FUNCTION "FC_GRP_43" : VOID
TITLE =GROUP =43
{ S7_language := '9(1) Angielski (Stany Zjednoczone)  11.01.2022  09:45:15' }
VERSION : 0.1


VAR_TEMP
  CL : "UDT_CABINET";	//CABINET LOCAL
  CR : "UDT_CABINET";	//CABINET REMOTE
  RelError : BOOL ;	//ERROR RELEASE
  RelErrorCL : BOOL ;	//ERROR RELEASE FROM CABINET LOCAL
  RelErrorCR : BOOL ;	//ERROR RELEASE FROM CABINET REMOTE
  RelControl : BOOL ;	//CONTROL RELEASE
  RelControlCL : BOOL ;	//CONTROL RELEASE FROM CABINET LOCAL
  RelControlCR : BOOL ;	//CONTROL RELEASE FROM CABINET REMOTE
  ErrorConfirm : BOOL ;	//ERROR CONFIRM
  AutoOn : BOOL ;	//AUTOMATIC ON
  AutoOff : BOOL ;	//AUTOMATIC OFF
  RelAuto : BOOL ;	//AUTOMATIC RELEASE
  LAMP_ON : BOOL ;
  TempSetpoint : REAL ;
END_VAR
BEGIN
NETWORK
TITLE =GLOBAL SIGNALS
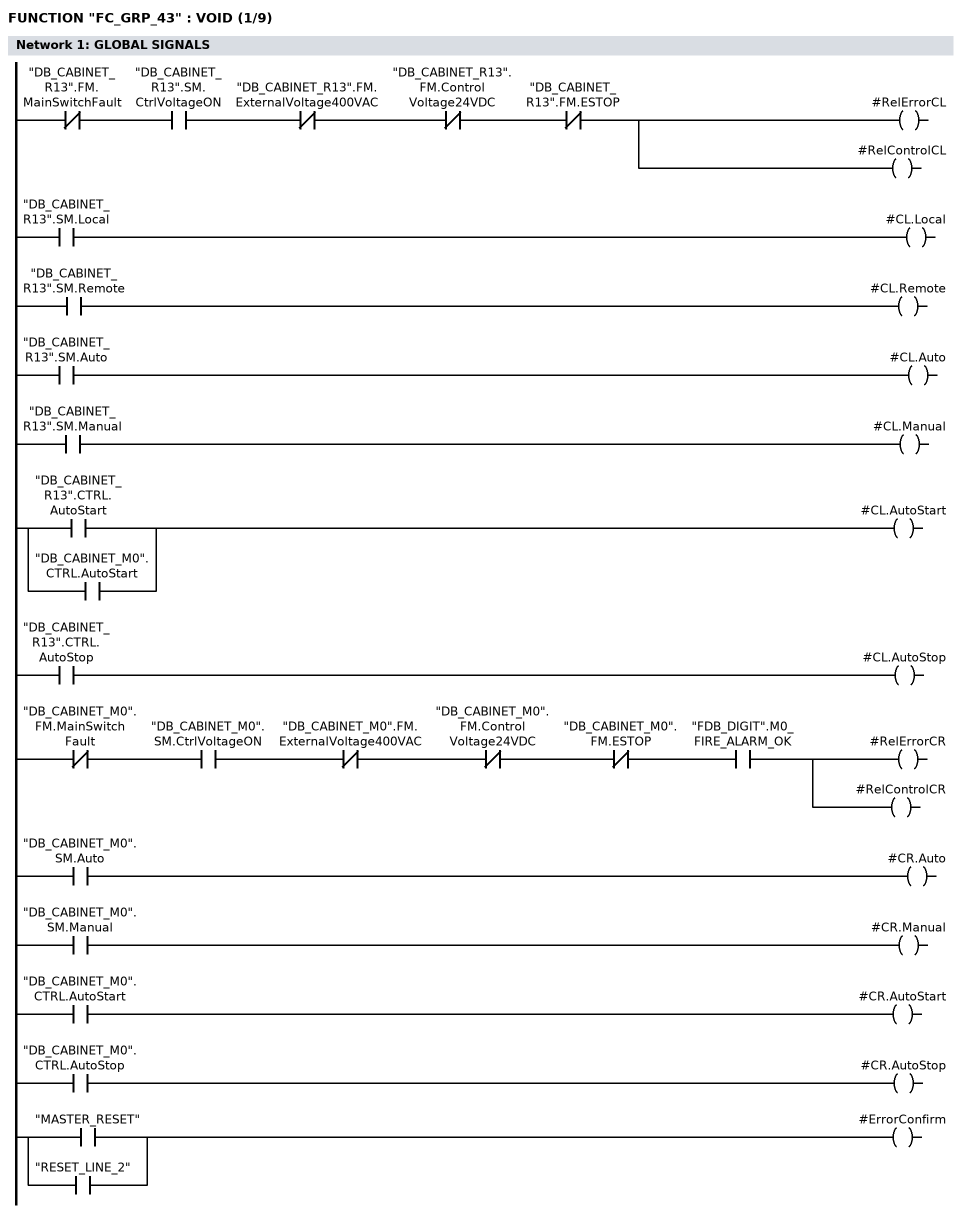
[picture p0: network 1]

//LOCAL
      UN    "DB_CABINET_R13".FM.MainSwitchFault;
      U     "DB_CABINET_R13".SM.CtrlVoltageON;
      UN    "DB_CABINET_R13".FM.ExternalVoltage400VAC;
      UN    "DB_CABINET_R13".FM.ControlVoltage24VDC;
      UN    "DB_CABINET_R13".FM.ESTOP;
      =     #RelErrorCL;
      =     #RelControlCL;

      U     "DB_CABINET_R13".SM.Local;
      =     #CL.Local;
      U     "DB_CABINET_R13".SM.Remote;
      =     #CL.Remote;
      U     "DB_CABINET_R13".SM.Auto;
      =     #CL.Auto;
      U     "DB_CABINET_R13".SM.Manual;
      =     #CL.Manual;
      U     "DB_CABINET_R13".CTRL.AutoStart;
      O     "DB_CABINET_M0".CTRL.AutoStart;
      =     #CL.AutoStart;
      U     "DB_CABINET_R13".CTRL.AutoStop;
      =     #CL.AutoStop;


//REMOTE
      UN    "DB_CABINET_M0".FM.MainSwitchFault;
      U     "DB_CABINET_M0".SM.CtrlVoltageON;
      UN    "DB_CABINET_M0".FM.ExternalVoltage400VAC;
      UN    "DB_CABINET_M0".FM.ControlVoltage24VDC;
//      UN    "DB_CABINET_M0".FM.ControlVoltage230VAC_MS
      UN    "DB_CABINET_M0".FM.ESTOP;
      U     "FDB_DIGIT".M0_FIRE_ALARM_OK;
      =     #RelErrorCR;
      =     #RelControlCR;

      U     "DB_CABINET_M0".SM.Auto;
      =     #CR.Auto;
      U     "DB_CABINET_M0".SM.Manual;
      =     #CR.Manual;
      U     "DB_CABINET_M0".CTRL.AutoStart;
      =     #CR.AutoStart;
      U     "DB_CABINET_M0".CTRL.AutoStop;
      =     #CR.AutoStop;


      U     "MASTER_RESET";
      O     "RESET_LINE_2";
      =     #ErrorConfirm;

NETWORK
TITLE =GLOBAL SIGNALS - GROUP GENERAL ERROR AND WARNING
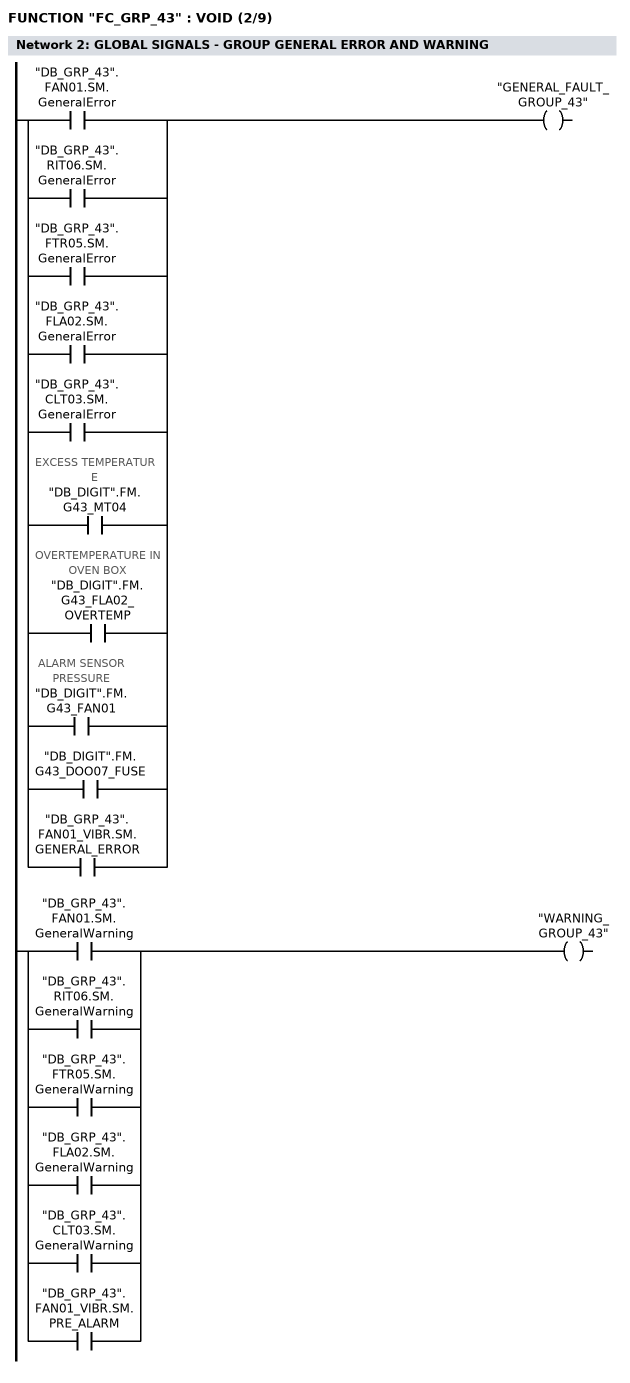
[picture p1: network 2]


      U     "DB_GRP_43".FAN01.SM.GeneralError;
      O     "DB_GRP_43".RIT06.SM.GeneralError;
      O     "DB_GRP_43".FTR05.SM.GeneralError;
      O     "DB_GRP_43".FLA02.SM.GeneralError;
      O     "DB_GRP_43".CLT03.SM.GeneralError;
      O     "DB_DIGIT".FM.G43_MT04; //EXCESS TEMPERATURE
      O     "DB_DIGIT".FM.G43_FLA02_OVERTEMP; //OVERTEMPERATURE IN OVEN BOX
      O     "DB_DIGIT".FM.G43_FAN01; //ALARM SENSOR PRESSURE
      O     "DB_DIGIT".FM.G43_DOO07_FUSE;
      O     "DB_GRP_43".FAN01_VIBR.SM.GENERAL_ERROR;
      =     "GENERAL_FAULT_GROUP_43";

      U     "DB_GRP_43".FAN01.SM.GeneralWarning;
      O     "DB_GRP_43".RIT06.SM.GeneralWarning;
      O     "DB_GRP_43".FTR05.SM.GeneralWarning;
      O     "DB_GRP_43".FLA02.SM.GeneralWarning;
      O     "DB_GRP_43".CLT03.SM.GeneralWarning;
      O     "DB_GRP_43".FAN01_VIBR.SM.PRE_ALARM;
      =     "WARNING_GROUP_43";


NETWORK
TITLE =RELEASE CONTROL
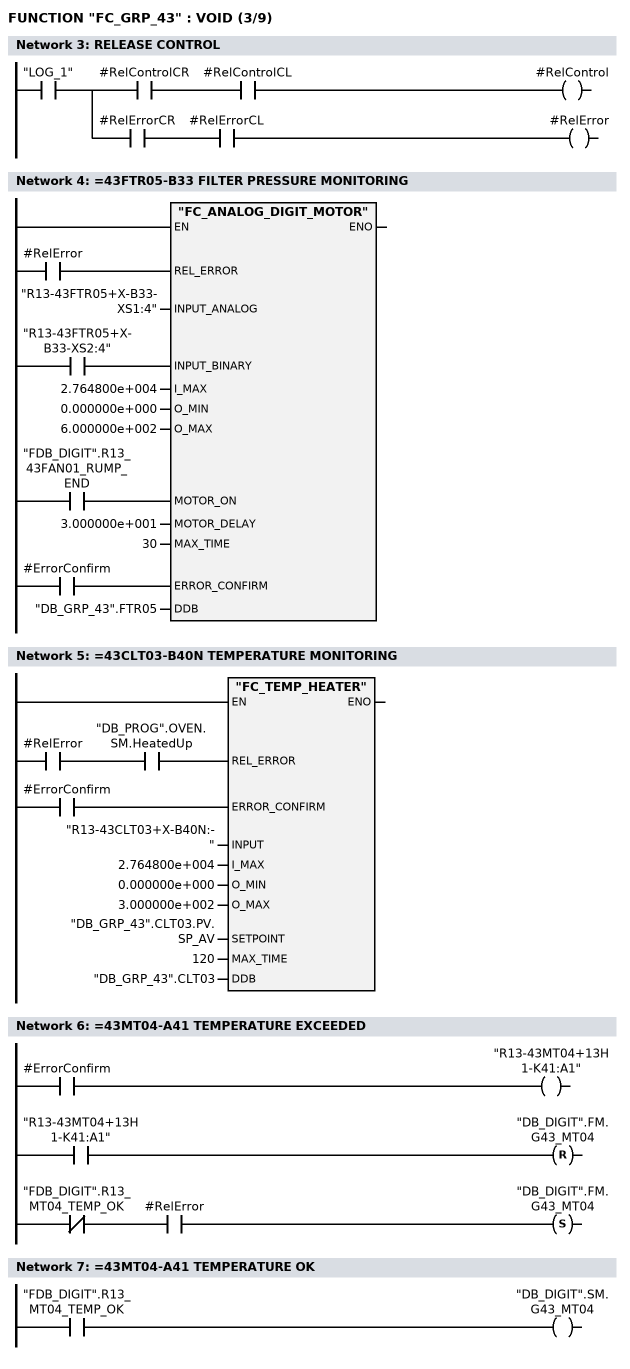
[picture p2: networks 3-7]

      U     "LOG_1";
      =     L     10.0;
      U     L     10.0;
      U     #RelControlCR;
      U     #RelControlCL;
      =     #RelControl;
      U     L     10.0;
      U     #RelErrorCR;
      U     #RelErrorCL;
      =     #RelError;
NETWORK
TITLE ==43FTR05-B33 FILTER PRESSURE MONITORING

      U     #RelError;
      =     L     10.0;
      BLD   103;
      U     "R13-43FTR05+X-B33-XS2:4";
      =     L     10.1;
      BLD   103;
      U     "FDB_DIGIT".R13_43FAN01_RUMP_END;
      =     L     10.2;
      BLD   103;
      U     #ErrorConfirm;
      =     L     10.3;
      BLD   103;
      CALL "FC_ANALOG_DIGIT_MOTOR" (
           REL_ERROR                := L     10.0,
           INPUT_ANALOG             := "R13-43FTR05+X-B33-XS1:4",
           INPUT_BINARY             := L     10.1,
           I_MAX                    := 2.764800e+004,
           O_MIN                    := 0.000000e+000,
           O_MAX                    := 6.000000e+002,
           MOTOR_ON                 := L     10.2,
           MOTOR_DELAY              := 3.000000e+001,
           MAX_TIME                 := 30,
           ERROR_CONFIRM            := L     10.3,
           DDB                      := "DB_GRP_43".FTR05);
      NOP   0;
NETWORK
TITLE ==43CLT03-B40N TEMPERATURE MONITORING

      U     #RelError;
      U     "DB_PROG".OVEN.SM.HeatedUp;
      =     L     10.0;
      BLD   103;
      U     #ErrorConfirm;
      =     L     10.1;
      BLD   103;
      CALL "FC_TEMP_HEATER" (
           REL_ERROR                := L     10.0,
           ERROR_CONFIRM            := L     10.1,
           INPUT                    := "R13-43CLT03+X-B40N:-",
           I_MAX                    := 2.764800e+004,
           O_MIN                    := 0.000000e+000,
           O_MAX                    := 3.000000e+002,
           SETPOINT                 := "DB_GRP_43".CLT03.PV.SP_AV,
           MAX_TIME                 := 120,
           DDB                      := "DB_GRP_43".CLT03);
      NOP   0;
NETWORK
TITLE ==43MT04-A41 TEMPERATURE EXCEEDED

      U     #ErrorConfirm;
      =     "R13-43MT04+13H1-K41:A1";
      U     "R13-43MT04+13H1-K41:A1";
      R     "DB_DIGIT".FM.G43_MT04;
      UN    "FDB_DIGIT".R13_MT04_TEMP_OK;
      U     #RelError;
      S     "DB_DIGIT".FM.G43_MT04;
      NOP   0;
NETWORK
TITLE ==43MT04-A41 TEMPERATURE OK

      U     "FDB_DIGIT".R13_MT04_TEMP_OK;
      =     "DB_DIGIT".SM.G43_MT04;
NETWORK
TITLE ==43DOO07-F1.1 ACCESS DOOR ERROR
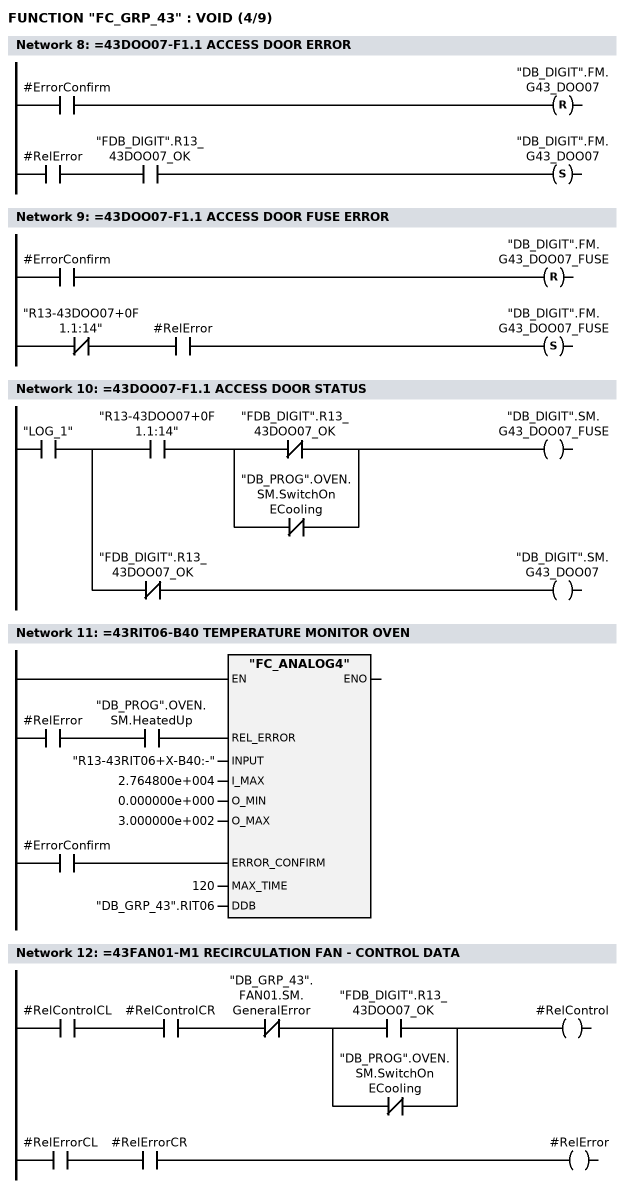
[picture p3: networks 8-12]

      U     #ErrorConfirm;
      R     "DB_DIGIT".FM.G43_DOO07;
      U     #RelError;
      U     "FDB_DIGIT".R13_43DOO07_OK;
      S     "DB_DIGIT".FM.G43_DOO07;
      NOP   0;
NETWORK
TITLE ==43DOO07-F1.1 ACCESS DOOR FUSE ERROR

      U     #ErrorConfirm;
      R     "DB_DIGIT".FM.G43_DOO07_FUSE;
      UN    "R13-43DOO07+0F1.1:14";
      U     #RelError;
      S     "DB_DIGIT".FM.G43_DOO07_FUSE;
      NOP   0;
NETWORK
TITLE ==43DOO07-F1.1 ACCESS DOOR STATUS

      U     "LOG_1";
      =     L     10.0;
      U     L     10.0;
      U     "R13-43DOO07+0F1.1:14";
      U(    ;
      ON    "FDB_DIGIT".R13_43DOO07_OK;
      ON    "DB_PROG".OVEN.SM.SwitchOnECooling;
      )     ;
      =     "DB_DIGIT".SM.G43_DOO07_FUSE;
      U     L     10.0;
      UN    "FDB_DIGIT".R13_43DOO07_OK;
      =     "DB_DIGIT".SM.G43_DOO07;
NETWORK
TITLE ==43RIT06-B40 TEMPERATURE MONITOR OVEN

      U     #RelError;
      U     "DB_PROG".OVEN.SM.HeatedUp;
      =     L     10.0;
      BLD   103;
      U     #ErrorConfirm;
      =     L     10.1;
      BLD   103;
      CALL "FC_ANALOG4" (
           REL_ERROR                := L     10.0,
           INPUT                    := "R13-43RIT06+X-B40:-",
           I_MAX                    := 2.764800e+004,
           O_MIN                    := 0.000000e+000,
           O_MAX                    := 3.000000e+002,
           ERROR_CONFIRM            := L     10.1,
           MAX_TIME                 := 120,
           DDB                      := "DB_GRP_43".RIT06);
      NOP   0;
NETWORK
TITLE ==43FAN01-M1 RECIRCULATION FAN - CONTROL DATA

      U     #RelControlCL;
      U     #RelControlCR;
      UN    "DB_GRP_43".FAN01.SM.GeneralError;
      U(    ;
      O     "FDB_DIGIT".R13_43DOO07_OK;
      ON    "DB_PROG".OVEN.SM.SwitchOnECooling;
      )     ;
      =     #RelControl;


      U     #RelErrorCL;
      U     #RelErrorCR;
      =     #RelError;

NETWORK
TITLE ==43FAN01-M1 RECIRCULATION FAN - AUTOMATIC MODE CONTROL SIGNALS
//2016.04.07 TC: CHANGED TEMPERATURE IN CMP FROM 91 TO 95 BECAUSE FAN WAS
//STOPPED AND STARTED 4 TIMES DURING OVEN'S STOPPING PROCEDURE - TEMPERATURE WAS
//GOING DOWN UNDER 90 oC AND UP ABOVE 91 oC. SOFT STARTER SHOULDN'T BE STARTED SO
//OFTEN
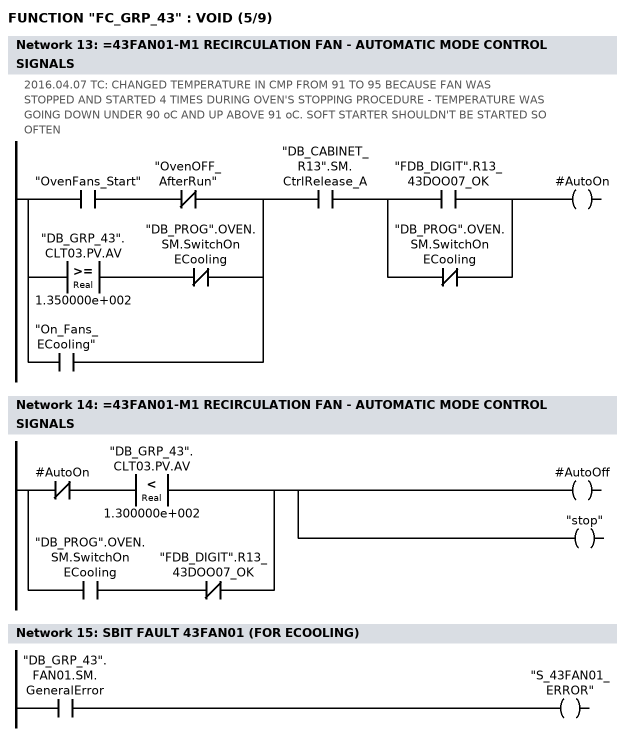
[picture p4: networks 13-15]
      U(    ;
      U     "OvenFans_Start";
      UN    "OvenOFF_AfterRun";
      O     ;
      U(    ;
      L     "DB_GRP_43".CLT03.PV.AV;
      L     1.350000e+002;
      >=R   ;
      )     ;
      UN    "DB_PROG".OVEN.SM.SwitchOnECooling;
      O     "On_Fans_ECooling";
      )     ;
      U     "DB_CABINET_R13".SM.CtrlRelease_A;
      U(    ;
      O     "FDB_DIGIT".R13_43DOO07_OK;
      ON    "DB_PROG".OVEN.SM.SwitchOnECooling;
      )     ;
      =     #AutoOn;
NETWORK
TITLE ==43FAN01-M1 RECIRCULATION FAN - AUTOMATIC MODE CONTROL SIGNALS

      UN    #AutoOn;
      U(    ;
      L     "DB_GRP_43".CLT03.PV.AV;
      L     1.300000e+002;
      <R    ;
      )     ;
      O     ;
      U     "DB_PROG".OVEN.SM.SwitchOnECooling;
      UN    "FDB_DIGIT".R13_43DOO07_OK;
      =     #AutoOff;
      =     "stop";
NETWORK
TITLE =SBIT FAULT 43FAN01 (FOR ECOOLING)

      U     "DB_GRP_43".FAN01.SM.GeneralError;
      =     "S_43FAN01_ERROR";
NETWORK
TITLE ==43FAN01-M1 RECIRCULATION FAN
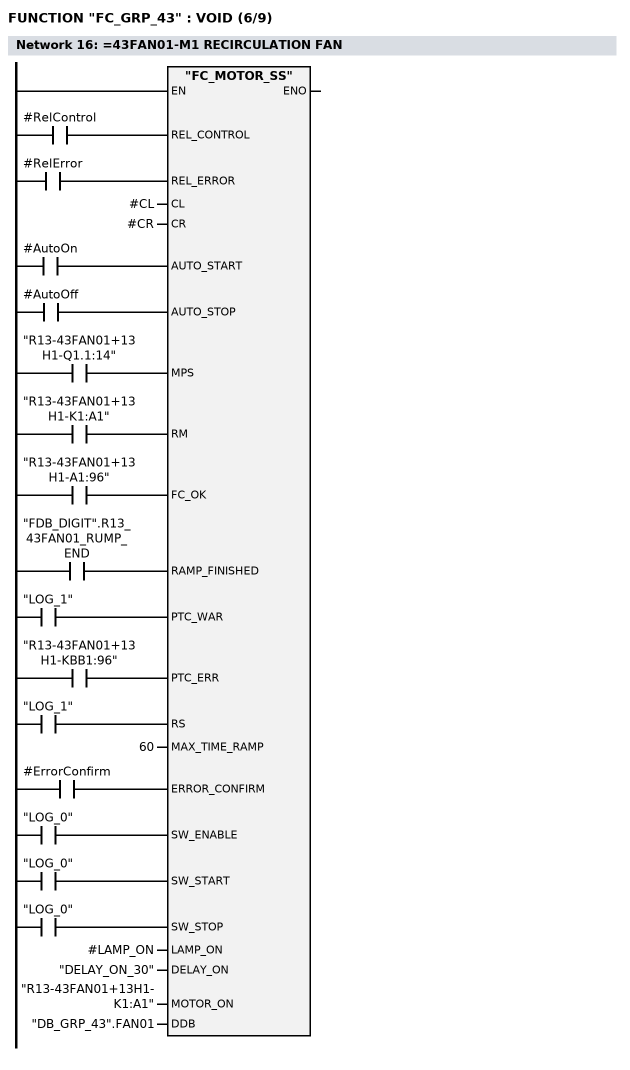
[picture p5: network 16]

      U     #RelControl;
      =     L     10.0;
      BLD   103;
      U     #RelError;
      =     L     10.1;
      BLD   103;
      U     #AutoOn;
      =     L     10.2;
      BLD   103;
      U     #AutoOff;
      =     L     10.3;
      BLD   103;
      U     "R13-43FAN01+13H1-Q1.1:14";
      =     L     10.4;
      BLD   103;
      U     "R13-43FAN01+13H1-K1:A1";
      =     L     10.5;
      BLD   103;
      U     "R13-43FAN01+13H1-A1:96";
      =     L     10.6;
      BLD   103;
      U     "FDB_DIGIT".R13_43FAN01_RUMP_END;
      =     L     10.7;
      BLD   103;
      U     "LOG_1";
      =     L     11.0;
      BLD   103;
      U     "R13-43FAN01+13H1-KBB1:96";
      =     L     11.1;
      BLD   103;
      U     "LOG_1";
      =     L     11.2;
      BLD   103;
      U     #ErrorConfirm;
      =     L     11.3;
      BLD   103;
      U     "LOG_0";
      =     L     11.4;
      BLD   103;
      U     "LOG_0";
      =     L     11.5;
      BLD   103;
      U     "LOG_0";
      =     L     11.6;
      BLD   103;
      CALL "FC_MOTOR_SS" (
           REL_CONTROL              := L     10.0,
           REL_ERROR                := L     10.1,
           CL                       := #CL,
           CR                       := #CR,
           AUTO_START               := L     10.2,
           AUTO_STOP                := L     10.3,
           MPS                      := L     10.4,
           RM                       := L     10.5,
           FC_OK                    := L     10.6,
           RAMP_FINISHED            := L     10.7,
           PTC_WAR                  := L     11.0,
           PTC_ERR                  := L     11.1,
           RS                       := L     11.2,
           MAX_TIME_RAMP            := 60,
           ERROR_CONFIRM            := L     11.3,
           SW_ENABLE                := L     11.4,
           SW_START                 := L     11.5,
           SW_STOP                  := L     11.6,
           LAMP_ON                  := #LAMP_ON,
           DELAY_ON                 := "DELAY_ON_30",
           MOTOR_ON                 := "R13-43FAN01+13H1-K1:A1",
           DDB                      := "DB_GRP_43".FAN01);
      NOP   0;
NETWORK
TITLE ==43FAN01-S32F RECIRCULATION FAN PRESSURE OK
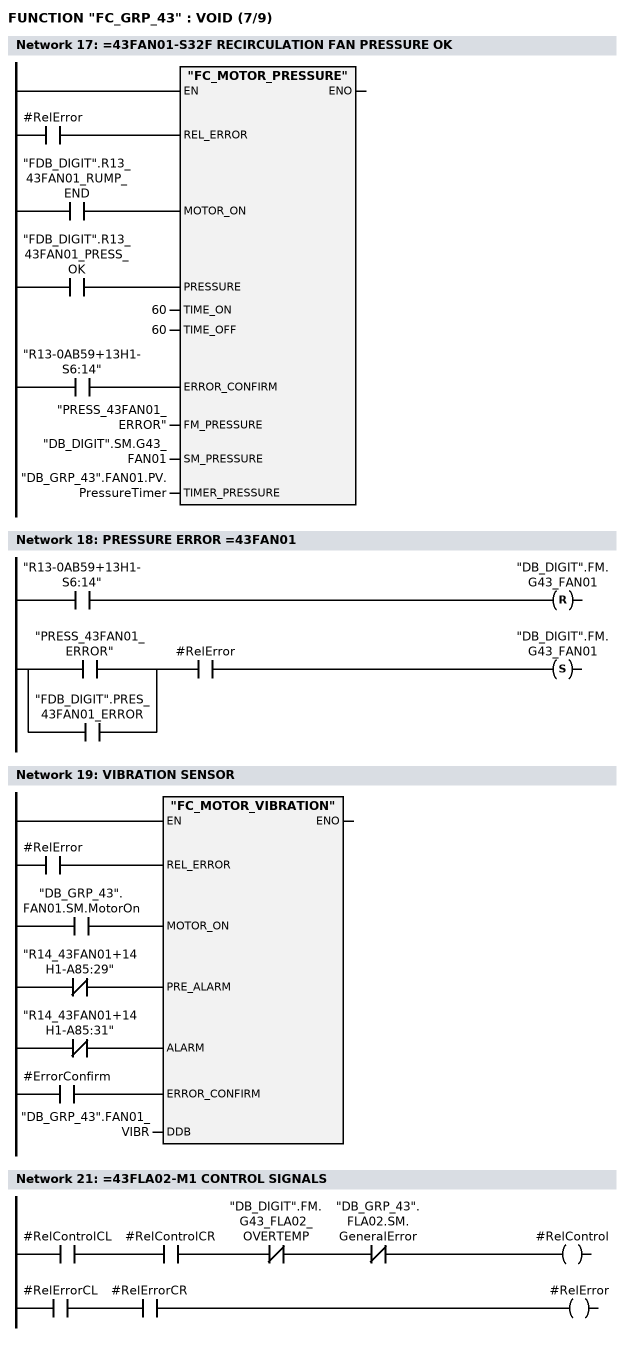
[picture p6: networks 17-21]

      U     #RelError;
      =     L     10.0;
      BLD   103;
      U     "FDB_DIGIT".R13_43FAN01_RUMP_END;
      =     L     10.1;
      BLD   103;
      U     "FDB_DIGIT".R13_43FAN01_PRESS_OK;
      =     L     10.2;
      BLD   103;
      U     "R13-0AB59+13H1-S6:14";
      =     L     10.3;
      BLD   103;
      CALL "FC_MOTOR_PRESSURE" (
           REL_ERROR                := L     10.0,
           MOTOR_ON                 := L     10.1,
           PRESSURE                 := L     10.2,
           TIME_ON                  := 60,
           TIME_OFF                 := 60,
           ERROR_CONFIRM            := L     10.3,
           FM_PRESSURE              := "PRESS_43FAN01_ERROR",
           SM_PRESSURE              := "DB_DIGIT".SM.G43_FAN01,
           TIMER_PRESSURE           := "DB_GRP_43".FAN01.PV.PressureTimer);
      NOP   0;
NETWORK
TITLE =PRESSURE ERROR =43FAN01

      U     "R13-0AB59+13H1-S6:14";
      R     "DB_DIGIT".FM.G43_FAN01;
      U(    ;
      O     "PRESS_43FAN01_ERROR";
      O     "FDB_DIGIT".PRES_43FAN01_ERROR;
      )     ;
      U     #RelError;
      S     "DB_DIGIT".FM.G43_FAN01;
      NOP   0;
NETWORK
TITLE =VIBRATION SENSOR

      U     #RelError;
      =     L     10.0;
      BLD   103;
      U     "DB_GRP_43".FAN01.SM.MotorOn;
      =     L     10.1;
      BLD   103;
      UN    "R14_43FAN01+14H1-A85:29";
      =     L     10.2;
      BLD   103;
      UN    "R14_43FAN01+14H1-A85:31";
      =     L     10.3;
      BLD   103;
      U     #ErrorConfirm;
      =     L     10.4;
      BLD   103;
      CALL "FC_MOTOR_VIBRATION" (
           REL_ERROR                := L     10.0,
           MOTOR_ON                 := L     10.1,
           PRE_ALARM                := L     10.2,
           ALARM                    := L     10.3,
           ERROR_CONFIRM            := L     10.4,
           DDB                      := "DB_GRP_43".FAN01_VIBR);
      NOP   0;
NETWORK
TITLE =************ 43FLA02 ****************

NETWORK
TITLE ==43FLA02-M1 CONTROL SIGNALS

      U     #RelControlCL;
      U     #RelControlCR;
      UN    "DB_DIGIT".FM.G43_FLA02_OVERTEMP;
      UN    "DB_GRP_43".FLA02.SM.GeneralError;
      =     #RelControl;


      U     #RelErrorCL;
      U     #RelErrorCR;
      =     #RelError;


NETWORK
TITLE ==43FLA02, CONTROL SIGNALS - AUTO_ON
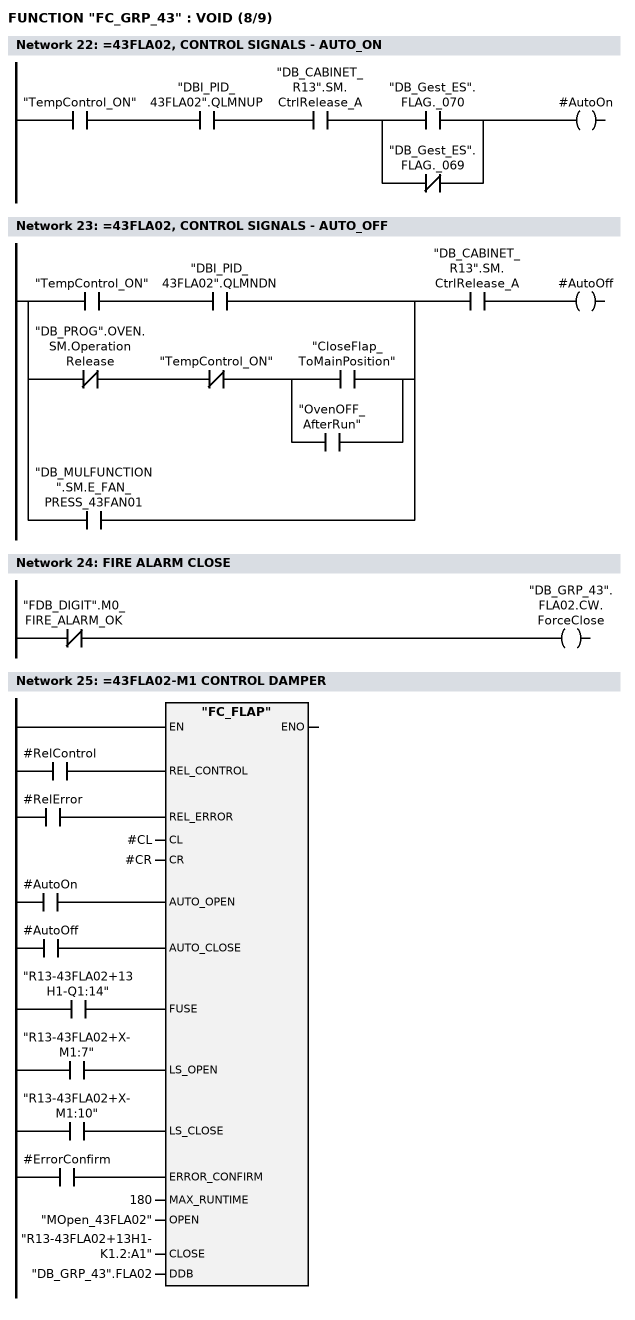
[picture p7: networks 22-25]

      U     "TempControl_ON";
      U     "DBI_PID_43FLA02".QLMNUP;
      U     "DB_CABINET_R13".SM.CtrlRelease_A;
      U(    ;
      O     "DB_Gest_ES".FLAG._070;
      ON    "DB_Gest_ES".FLAG._069;
      )     ;
      =     #AutoOn;
NETWORK
TITLE ==43FLA02, CONTROL SIGNALS - AUTO_OFF

      U(    ;
      U     "TempControl_ON";
      U     "DBI_PID_43FLA02".QLMNDN;
      O     ;
      UN    "DB_PROG".OVEN.SM.OperationRelease;
      UN    "TempControl_ON";
      U(    ;
      O     "CloseFlap_ToMainPosition";
      O     "OvenOFF_AfterRun";
      )     ;
      O     "DB_MULFUNCTION".SM.E_FAN_PRESS_43FAN01;
      )     ;
      U     "DB_CABINET_R13".SM.CtrlRelease_A;
      =     #AutoOff;
NETWORK
TITLE =FIRE ALARM CLOSE

      UN    "FDB_DIGIT".M0_FIRE_ALARM_OK;
      =     "DB_GRP_43".FLA02.CW.ForceClose;
NETWORK
TITLE ==43FLA02-M1 CONTROL DAMPER



      U     #RelControl;
      =     L     10.0;
      BLD   103;
      U     #RelError;
      =     L     10.1;
      BLD   103;
      U     #AutoOn;
      =     L     10.2;
      BLD   103;
      U     #AutoOff;
      =     L     10.3;
      BLD   103;
      U     "R13-43FLA02+13H1-Q1:14";
      =     L     10.4;
      BLD   103;
      U     "R13-43FLA02+X-M1:7";
      =     L     10.5;
      BLD   103;
      U     "R13-43FLA02+X-M1:10";
      =     L     10.6;
      BLD   103;
      U     #ErrorConfirm;
      =     L     10.7;
      BLD   103;
      CALL "FC_FLAP" (
           REL_CONTROL              := L     10.0,
           REL_ERROR                := L     10.1,
           CL                       := #CL,
           CR                       := #CR,
           AUTO_OPEN                := L     10.2,
           AUTO_CLOSE               := L     10.3,
           FUSE                     := L     10.4,
           LS_OPEN                  := L     10.5,
           LS_CLOSE                 := L     10.6,
           ERROR_CONFIRM            := L     10.7,
           MAX_RUNTIME              := 180,
           OPEN                     := "MOpen_43FLA02",
           CLOSE                    := "R13-43FLA02+13H1-K1.2:A1",
           DDB                      := "DB_GRP_43".FLA02);
      NOP   0;
NETWORK
TITLE =MANUAL INTERLOCKS - OPEN 43FLA02
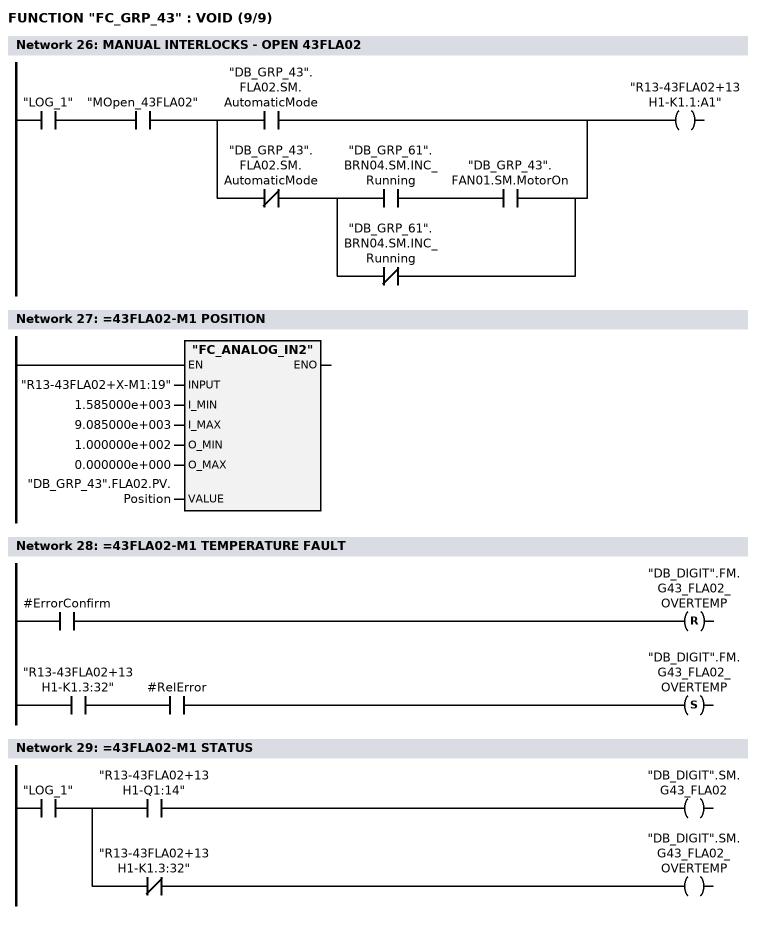
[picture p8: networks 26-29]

      U     "LOG_1";
      U     "MOpen_43FLA02";
      U(    ;
      O     "DB_GRP_43".FLA02.SM.AutomaticMode;
      O     ;
      UN    "DB_GRP_43".FLA02.SM.AutomaticMode;
      U(    ;
      U     "DB_GRP_61".BRN04.SM.INC_Running;
      U     "DB_GRP_43".FAN01.SM.MotorOn;
      ON    "DB_GRP_61".BRN04.SM.INC_Running;
      )     ;
      )     ;
      =     "R13-43FLA02+13H1-K1.1:A1";
NETWORK
TITLE ==43FLA02-M1 POSITION

      CALL "FC_ANALOG_IN2" (
           INPUT                    := "R13-43FLA02+X-M1:19",
           I_MIN                    := 1.585000e+003,
           I_MAX                    := 9.085000e+003,
           O_MIN                    := 1.000000e+002,
           O_MAX                    := 0.000000e+000,
           VALUE                    := "DB_GRP_43".FLA02.PV.Position);
      NOP   0;
NETWORK
TITLE ==43FLA02-M1 TEMPERATURE FAULT

      U     #ErrorConfirm;
      R     "DB_DIGIT".FM.G43_FLA02_OVERTEMP;
      U     "R13-43FLA02+13H1-K1.3:32";
      U     #RelError;
      S     "DB_DIGIT".FM.G43_FLA02_OVERTEMP;
      NOP   0;
NETWORK
TITLE ==43FLA02-M1 STATUS

      U     "LOG_1";
      =     L     10.0;
      U     L     10.0;
      U     "R13-43FLA02+13H1-Q1:14";
      =     "DB_DIGIT".SM.G43_FLA02;
      U     L     10.0;
      UN    "R13-43FLA02+13H1-K1.3:32";
      =     "DB_DIGIT".SM.G43_FLA02_OVERTEMP;
NETWORK
TITLE =END

END_FUNCTION

